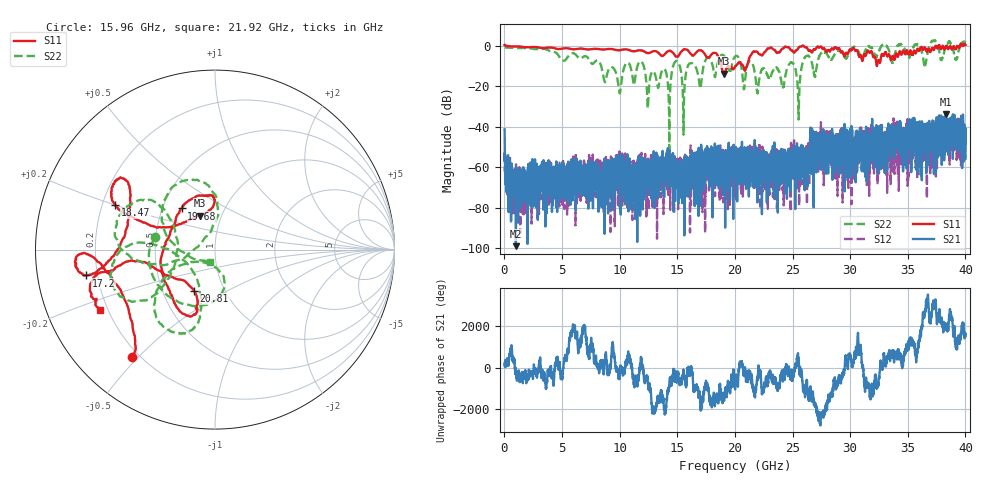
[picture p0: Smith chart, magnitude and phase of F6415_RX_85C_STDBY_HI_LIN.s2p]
!Keysight Technologies,N5245B,MY52451815,A.15.70.20
!Date: Wednesday, April 17, 2024 16:19:00
!Correction: S33(C  2-Port  )
!S43(C  2-Port  )
!S34(C  2-Port  )
!S44(C  2-Port  )
!S2P File: Measurements: S33, S43, S34, S44:
# Hz S  RI  R 50
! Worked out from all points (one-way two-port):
!   4000 points, 10 MHz to 40 GHz, reference 50 ohm
!   highest |S21| = -33.79 dB at 38.3 GHz (marker M1); lowest = -99.1 dB at 990 MHz (marker M2)
!   lowest |S11| = -13.7 dB at 19.06 GHz (marker M3), VSWR 1.52, Z = 39.5 + j15.7 ohm
!   |S11| at or under -10 dB: 18.82 GHz to 20.03 GHz (1.215 GHz wide, 6.26 % of centre); 20.71 GHz to 21.03 GHz (318.3 MHz wide, 1.53 % of centre)
!   |S22| runs from -54.3 to 2.7 dB; largest |S21 - S12| = 0.029
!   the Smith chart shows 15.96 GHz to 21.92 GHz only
!   S11 on the Smith chart (normalised r, x): 15.96 GHz: 0.17, -0.48; 17.2 GHz: 0.16, -0.10; 18.47 GHz: 0.25, +0.20; 19.68 GHz: 0.63, +0.31; 20.81 GHz: 0.72, -0.35; 21.92 GHz: 0.17, -0.24
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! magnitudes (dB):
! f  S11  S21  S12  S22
! 10 MHz  0.4  -41.3  -56.8  -0.8
! 990 MHz  -0.3  -99.1  -75.2  -1.0
! 6.68 GHz  -1.3  -72.8  -71.2  -6.0
! 13.34 GHz  -3.4  -57.9  -56.9  -20.5
! 14.32 GHz  -2.4  -60.9  -60.2  -33.5
! 14.95 GHz  -5.3  -61.1  -70.4  -7.4
! 15.56 GHz  -1.7  -58.6  -63.2  -32.5
! 15.96 GHz  -2.4  -59.5  -59.8  -9.3
! 17.2 GHz  -2.7  -59.6  -73.4  -12.4
! 18.47 GHz  -4.3  -57.5  -54.1  -9.2
! 19.06 GHz  -13.7  -63.0  -62.0  -4.9
! 19.68 GHz  -10.6  -64.3  -53.7  -10.7
! 20.01 GHz  -10.1  -55.3  -55.7  -5.3
! 20.81 GHz  -11.8  -68.0  -54.6  -21.2
! 21.35 GHz  -4.7  -53.3  -54.2  -7.5
! 21.92 GHz  -2.8  -57.4  -56.4  -22.6
! 24.92 GHz  -2.2  -57.9  -52.3  -8.1
! 25.52 GHz  -0.9  -53.8  -58.9  -36.4
! 26.67 GHz  -3.1  -46.8  -44.2  -8.3
! 33.34 GHz  -4.2  -44.1  -51.3  -1.8
! 38.3 GHz  -0.4  -33.8  -38.9  0.5
! 40 GHz  0.4  -48.2  -48.5  1.7
